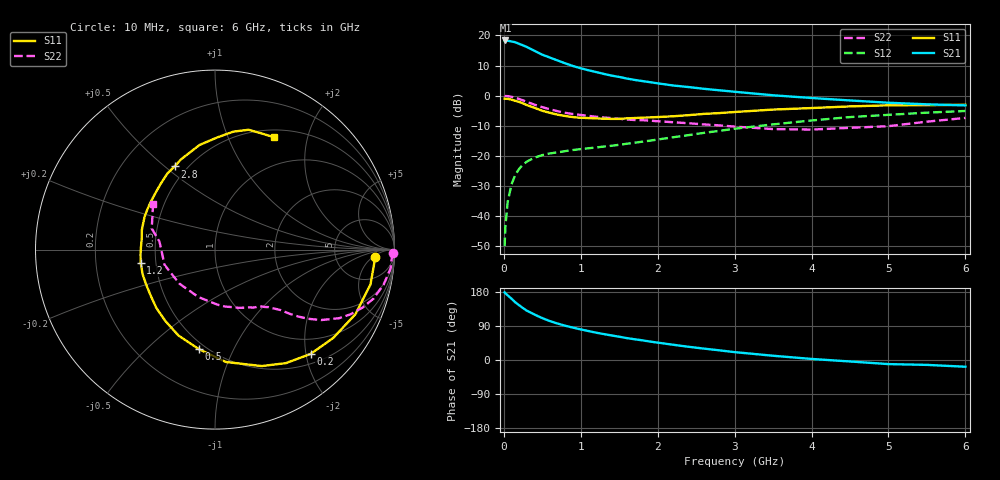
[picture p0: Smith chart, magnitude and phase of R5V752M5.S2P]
! SIEMENS Small Signal Semiconductors
! BFR183
! Si NPN RF Bipolar Junction Transistor in SOT23
! VCE = 0.75 V  IC = 2.5 mA
! Common Emitter S-Parameters:  May  1996
# GHz  S  MA  R  50
!  f  S11  S21  S12  S22
! GHz  MAG  ANG  MAG  ANG  MAG  ANG  MAG  ANG
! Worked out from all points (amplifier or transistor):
!   36 points, 10 MHz to 6 GHz, reference 50 ohm
!   highest |S21| = 18.3 dB at 20 MHz (marker M1)
!   |S21| within 3 dB of that: start of sweep to 364.3 MHz
!   unconditionally stable (mu >= 1): 1.267 GHz to 3.177 GHz
!   at 250 MHz: K = 0.27, MSG = 19.8 dB, |S12| = -22.8 dB
!   at 1.4 GHz: K = 1.06, MAG = 10.1 dB, |S12| = -16.6 dB
!   at 6 GHz: K = 0.96, MSG = 0.9 dB, |S12| = -5.1 dB
!   S11 on the Smith chart (normalised r, x): 10 MHz: 15, -6; 200 MHz: 0.68, -2.09; 500 MHz: 0.46, -0.74; 1.2 GHz: 0.41, -0.08; 2.8 GHz: 0.43, +0.54; 6 GHz: 0.60, +1.49
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0.01  0.8942 -2.6  8.143 178.5  0.0032 91.4  0.9926 -1.1
0.02  0.8903 -5.0  8.253 176.1  0.0067 84.6  0.9866 -2.4
0.05  0.8878 -12.6  8.159 170.6  0.0173 82.5  0.9839 -6.1
0.1  0.8613 -24.7  7.947 161.7  0.034 76.8  0.9594 -11.8
0.15  0.8222 -36.8  7.7 152.0  0.0492 69.6  0.9234 -17.3
0.2  0.7883 -47.5  7.239 144.4  0.0614 64.5  0.8826 -21.5
0.25  0.7454 -58.1  6.836 136.8  0.0724 59.8  0.8371 -25.5
0.3  0.6988 -68.2  6.421 130.0  0.081 56.1  0.7907 -28.9
0.4  0.6287 -84.6  5.544 119.8  0.094 50.0  0.7096 -33.6
0.5  0.5626 -99.0  4.792 110.5  0.1037 45.9  0.6466 -36.6
0.6  0.5203 -113.0  4.288 102.6  0.1106 43.4  0.5951 -38.8
0.7  0.4851 -124.6  3.837 96.1  0.1153 42.0  0.5534 -40.5
0.8  0.4612 -135.1  3.437 90.3  0.1207 41.1  0.5206 -41.7
1.1  0.4261 -161.2  2.645 76.4  0.1345 40.9  0.4631 -45.1
1.2  0.4206 -169.6  2.468 72.1  0.1386 41.3  0.4486 -46.3
1.6  0.4221 164.9  1.927 57.8  0.1598 44.2  0.4044 -51.5
2.2  0.4562 137.3  1.479 40.3  0.2045 46.5  0.3636 -62.9
2.8  0.5153 115.9  1.231 25.5  0.2613 44.9  0.3225 -79.9
3.5  0.5893 98.4  1.017 11.2  0.3348 38.8  0.2798 -109.5
4.5  0.6655 81.1  0.835 -3.9  0.4427 26.6  0.2936 -163.1
5.5  0.6978 67.7  0.72 -12.9  0.5243 13.5  0.3715 161.6
6  0.7077 62.1  0.691 -17.8  0.5588 5.2  0.4285 143.6
